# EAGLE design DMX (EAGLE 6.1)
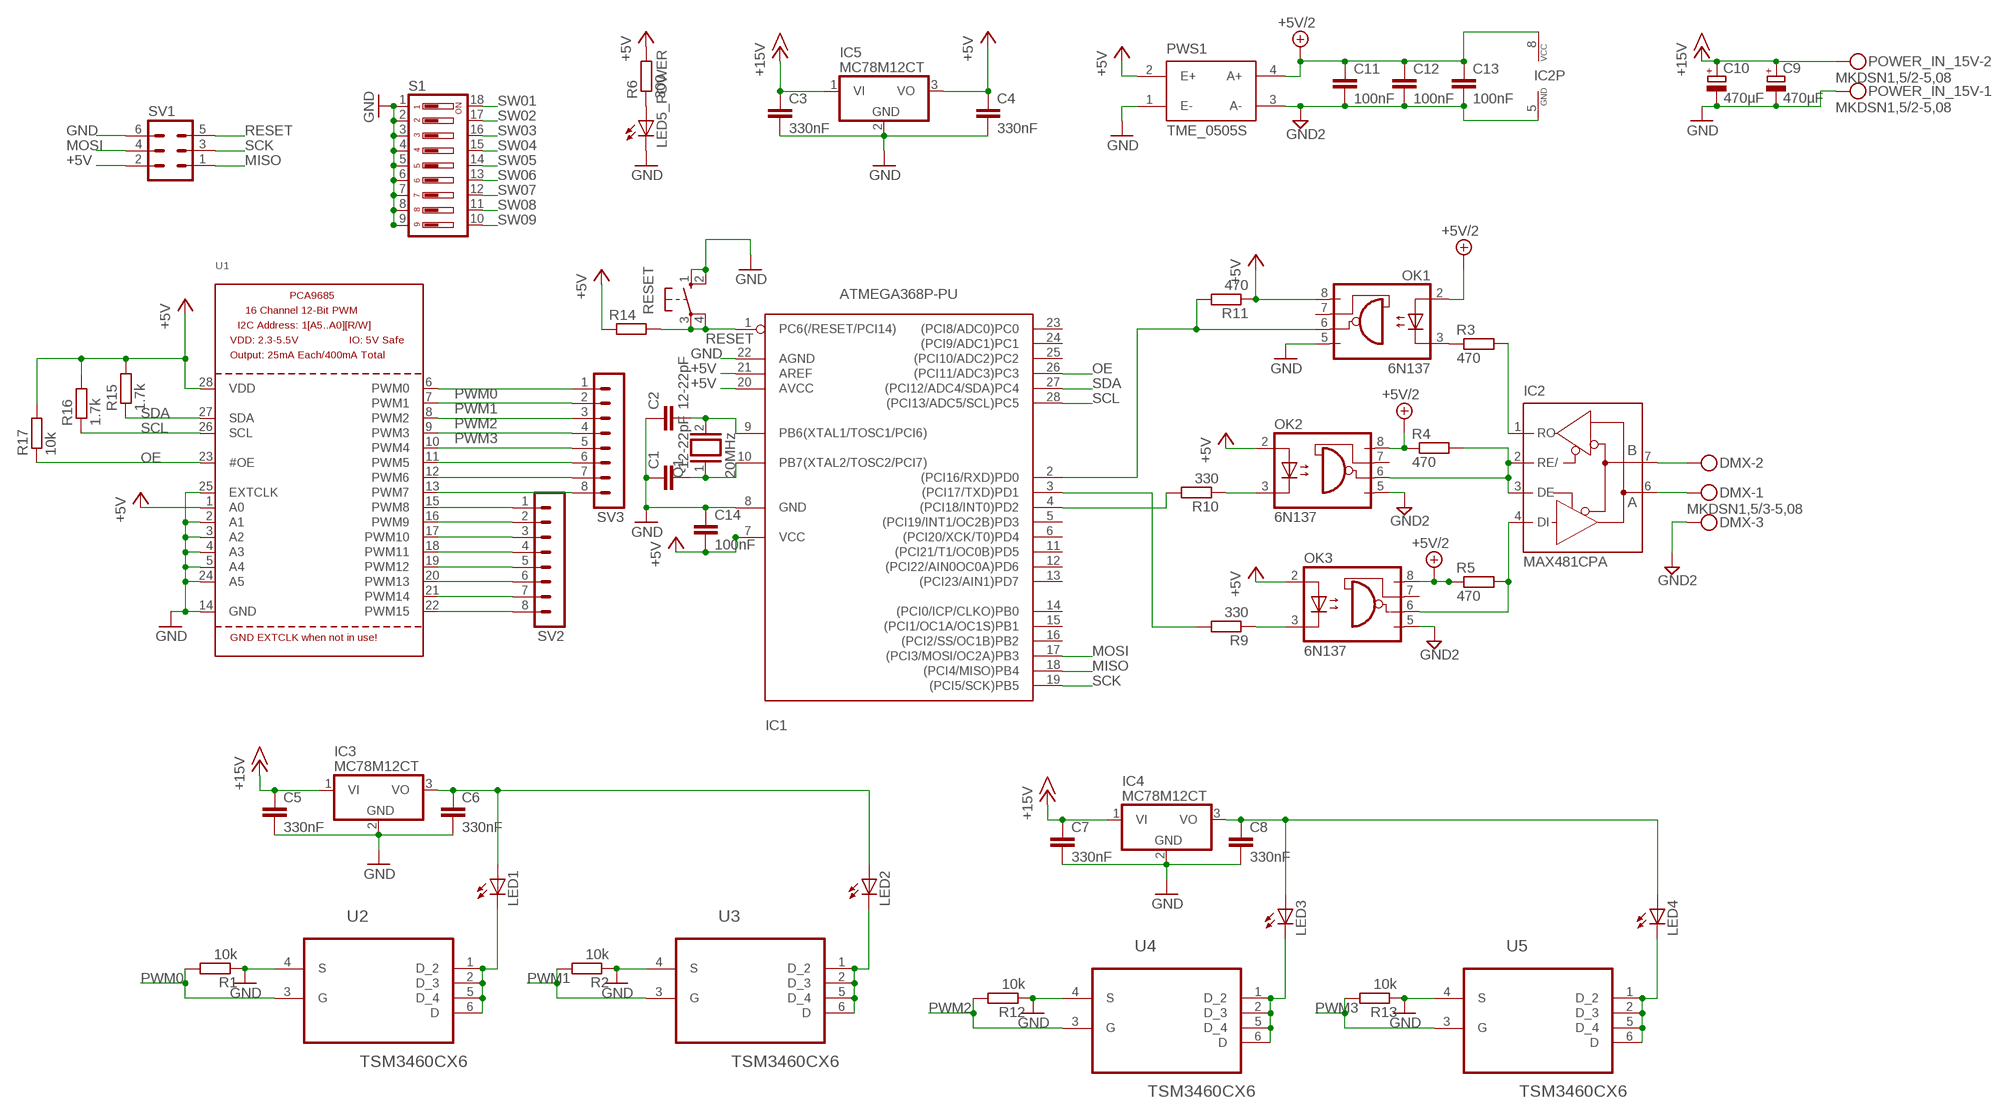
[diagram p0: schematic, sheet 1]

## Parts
C1  12-22pF  C-EU025-025X050  [C025-025X050]
C2  12-22pF  C-EU025-025X050  [C025-025X050]
C3  330nF  C-EU050-025X075  [C050-025X075]
C4  330nF  C-EU050-025X075  [C050-025X075]
C5  330nF  C-EU050-025X075  [C050-025X075]
C6  330nF  C-EU050-025X075  [C050-025X075]
C7  330nF  C-EU050-025X075  [C050-025X075]
C8  330nF  C-EU050-025X075  [C050-025X075]
C9  470µF  CPOL-EUE5-10.5  [E5-10,5]
C10  470µF  CPOL-EUE5-10.5  [E5-10,5]
C11  100nF  C-EU050-025X075  [C050-025X075]
C12  100nF  C-EU050-025X075  [C050-025X075]
C13  100nF  C-EU050-025X075  [C050-025X075]
C14  100nF  C-EU050-025X075  [C050-025X075]
DMX  MKDSN1,5/3-5,08  [MKDSN1,5/3-5,08]
IC1  ATMEGA368P-PU  ATMEGA168-20P  [DIL28-3]
IC2  MAX481CPA  [DIL08]
IC3  MC78M12CT  [TO220V]
IC4  MC78M12CT  [TO220V]
IC5  MC78M12CT  [TO220V]
LED1  LED5MM  [LED5MM]
LED2  LED5MM  [LED5MM]
LED3  LED5MM  [LED5MM]
LED4  LED5MM  [LED5MM]
LED5_POWER  LED5MM  [LED5MM]
OK1  6N137  [DIL08]
OK2  6N137  [DIL08]
OK3  6N137  [DIL08]
POWER_IN_15V  MKDSN1,5/2-5,08  [MKDSN1,5/2-5,08]
PWS1  TME_0505S  [TMEXXXXS]
Q1  20MHz  XTAL/S  [QS]
R1  10k  R-EU_0207/7  [0207/7]
R2  10k  R-EU_0207/7  [0207/7]
R3  470  R-EU_0207/7  [0207/7]
R4  470  R-EU_0207/7  [0207/7]
R5  470  R-EU_0207/7  [0207/7]
R6  300  R-EU_0204/7  [0204/7]
R9  330  R-EU_0207/7  [0207/7]
R10  330  R-EU_0207/7  [0207/7]
R11  470  R-EU_0207/7  [0207/7]
R12  10k  R-EU_0207/7  [0207/7]
R13  10k  R-EU_0207/7  [0207/7]
R14  R-EU_0204/7  [0204/7]
R15  1.7k  R-EU_0204/7  [0204/7]
R16  1.7k  R-EU_0204/7  [0204/7]
R17  10k  R-EU_0204/7  [0204/7]
RESET  10-XX  [B3F-10XX]
S1  DP09  [DP-09]
SV1  MA03-2  [MA03-2]
SV2  MA08-1  [MA08-1]
SV3  MA08-1  [MA08-1]
U1  PCA9685  [TSSOP28]
U2  TSM3460CX6  [SOT95P280X120-6N]
U3  TSM3460CX6  [SOT95P280X120-6N]
U4  TSM3460CX6  [SOT95P280X120-6N]
U5  TSM3460CX6  [SOT95P280X120-6N]

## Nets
+5V: C4.1 C14.2 IC1.7(VCC) IC1.20(AVCC) IC1.21(AREF) IC5.3(VO) OK1.8(VCC) OK2.2(A) OK3.2(A) PWS1.2(E+) R6.2 R11.1 R14.1 R15.2 R16.2 R17.2 SV1.2 U1.1(A0) U1.28(VDD)
+5V/2: C11.1 C12.1 C13.1 IC2.8(VCC) OK1.2(A) OK2.8(VCC) OK3.8(VCC) PWS1.4(A+) R4.1 R5.1
+15V: C3.1 C5.1 C7.1 C9.+ C10.+ IC3.1(VI) IC4.1(VI) IC5.1(VI) POWER_IN_15V.2
GND: C1.1 C2.1 C3.2 C4.2 C5.2 C6.2 C7.2 C8.2 C9.- C10.- C14.1 IC1.8(GND) IC1.22(AGND) IC3.2(GND) IC4.2(GND) IC5.2(GND) LED5_POWER.K(C) OK1.5(GND) POWER_IN_15V.1 PWS1.1(E-) R1.1 R2.1 R12.1 R13.1 RESET.1(S) RESET.2(S1) S1.1 S1.2 S1.3 S1.4 S1.5 S1.6 S1.7 S1.8 S1.9 SV1.6 U1.2(A1) U1.3(A2) U1.4(A3) U1.5(A4) U1.14(GND) U1.24(A5) U1.25(EXTCLK) U2.4(S) U3.4(S) U4.4(S) U5.4(S)
GND2: C11.2 C12.2 C13.2 DMX.3 IC2.5(GND) OK2.5(GND) OK3.5(GND) PWS1.3(A-)
MISO: IC1.18((PCI4/MISO)PB4) SV1.1
MOSI: IC1.17((PCI3/MOSI/OC2A)PB3) SV1.4
N$1: OK1.3(C) R3.1
N$2: IC2.1(RO) R3.2
N$3: IC2.2(RE/) IC2.3(DE) OK2.6(VO) R4.2
N$4: IC2.4(DI) OK3.6(VO) R5.2
N$5: OK3.3(C) R9.1
N$6: OK2.3(C) R10.1
N$7: IC1.2((PCI16/RXD)PD0) OK1.6(VO) R11.2
N$8: IC1.4((PCI18/INT0)PD2) R10.2
N$9: IC1.3((PCI17/TXD)PD1) R9.2
N$10: DMX.2 IC2.7(B)
N$11: DMX.1 IC2.6(A)
N$12: C6.1 IC3.3(VO) LED1.A LED2.A
N$13: LED3.K(C) U4.1(D_2) U4.2(D_3) U4.5(D_4) U4.6(D)
N$14: C8.1 IC4.3(VO) LED3.A LED4.A
N$15: LED1.K(C) U2.1(D_2) U2.2(D_3) U2.5(D_4) U2.6(D)
N$16: LED4.K(C) U5.1(D_2) U5.2(D_3) U5.5(D_4) U5.6(D)
N$17: LED2.K(C) U3.1(D_2) U3.2(D_3) U3.5(D_4) U3.6(D)
N$18: C1.2 IC1.10(PB7(XTAL2/TOSC2/PCI7)) Q1.1
N$19: C2.2 IC1.9(PB6(XTAL1/TOSC1/PCI6)) Q1.2
N$20: LED5_POWER.A R6.1
N$22: SV3.5 U1.10(PWM4)
N$23: SV3.6 U1.11(PWM5)
N$24: SV3.7 U1.12(PWM6)
N$25: SV3.8 U1.13(PWM7)
N$26: SV2.1 U1.15(PWM8)
N$27: SV2.2 U1.16(PWM9)
N$28: SV2.3 U1.17(PWM10)
N$29: SV2.4 U1.18(PWM11)
N$30: SV2.5 U1.19(PWM12)
N$31: SV2.6 U1.20(PWM13)
N$32: SV2.7 U1.21(PWM14)
N$33: SV2.8 U1.22(PWM15)
OE: IC1.26((PCI11/ADC3)PC3) R17.1 U1.23(#OE)
PWM0: R1.2 SV3.1 U1.6(PWM0) U2.3(G)
PWM1: R2.2 SV3.2 U1.7(PWM1) U3.3(G)
PWM2: R12.2 SV3.3 U1.8(PWM2) U4.3(G)
PWM3: R13.2 SV3.4 U1.9(PWM3) U5.3(G)
RESET: IC1.1(PC6(/RESET/PCI14)) R14.2 RESET.3(P) RESET.4(P1) SV1.5
SCK: IC1.19((PCI5/SCK)PB5) SV1.3
SCL: IC1.28((PCI13/ADC5/SCL)PC5) R16.1 U1.26(SCL)
SDA: IC1.27((PCI12/ADC4/SDA)PC4) R15.1 U1.27(SDA)
SW01: S1.18
SW02: S1.17
SW03: S1.16
SW04: S1.15
SW05: S1.14
SW06: S1.13
SW07: S1.12
SW08: S1.11
SW09: S1.10
Unconnected: IC1.5((PCI19/INT1/OC2B)PD3) IC1.6((PCI20/XCK/T0)PD4) IC1.11((PCI21/T1/OC0B)PD5) IC1.12((PCI22/AIN0OC0A)PD6) IC1.13((PCI23/AIN1)PD7) IC1.14((PCI0/ICP/CLKO)PB0) IC1.15((PCI1/OC1A/OC1S)PB1) IC1.16((PCI2/SS/OC1B)PB2) IC1.23((PCI8/ADC0)PC0) IC1.24((PCI9/ADC1)PC1) IC1.25((PCI10/ADC2)PC2) OK1.7(VE) OK2.7(VE) OK3.7(VE)

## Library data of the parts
C1-C8 C11-C14 = rcl:C-EU: CAPACITOR, European symbol
C9 C10 = rcl:CPOL-EU: POLARIZED CAPACITOR, European symbol
DMX = con-phoenix-508:MKDSN1,5/3-5,08: MKDSN 1,5/ 3-5,08 Printklemme Nennstrom: 13,5 A Nennspannung: 250 V Rastermaß: 5,08 mm Polzahl: 3 Anschlussart: Schraubanschluss Montage: Löten Anschlussrichtung Leiter/Platine: 0 ° Artikelnummer: 1729131 Source: http://eshop.phoenixcontact.com .. 1729131.pdf; MPN: SMKDSN1,5/3-5,08; OC_FARNELL: 1792904; OC_NEWARK: 70R0299
IC1 = adafruit:ATMEGA168*P: MICROCONTROLLER 16 kBytes FLASH 1 kBytes SRAM 512 Bytes EEPROM USART 8-channel 10 bit ADC
IC2 = maxim:MAX481CPA: RS485 TRANSEIVER; MPN: MAX485; OC_FARNELL: unknown; OC_NEWARK: 99K3445
IC3-IC5 = linear:MC78M: 500 mA Positive Voltage Regulators Source: Data sheet
LED1-LED4 LED5_POWER = led:LED: LED
OK1-OK3 = optocoupler:6N137: MOTOROLA OPTO COUPLER; MPN: 6N137; OC_FARNELL: 1328376; OC_NEWARK: 52M1895
POWER_IN_15V = con-phoenix-508:MKDSN1,5/2-5,08: MKDSN 1,5/ 2-5,08 Printklemme; MPN: MKDSN 1,5/2-5.08; OC_FARNELL: 1792903; OC_NEWARK: 30M2397
PWS1 = traco-electronic:TME_*S: DC/DC Konverter 1 Watt Source: http://www.tracopower.com/datasheet_g/tme-d.pdf; MPN: TME 0505S; OC_FARNELL: 1007538; OC_NEWARK: 51R5321
Q1 = special:XTAL/S: CRYSTAL
R1-R6 R9-R17 = rcl:R-EU_: RESISTOR, European symbol
RESET = switch-omron:10-XX: OMRON SWITCH; MPN: B3F-1000; OC_FARNELL: 176432; OC_NEWARK: 36M3542
S1 = switch-dil:DP09: DIL/CODE SWITCH; MPN: MCDP09; OC_FARNELL: 1522007; OC_NEWARK: 74M2979
SV1 = con-lstb:MA03-2: PIN HEADER; OC_FARNELL: unknown; OC_NEWARK: unknown
SV2 SV3 = con-lstb:MA08-1: PIN HEADER; OC_FARNELL: unknown; OC_NEWARK: unknown
U1 = adafruit:PCA9685: PCA9685 - 16 Channel 12-Bit I2C PWM Controller 5.0V tolerant 16 channel, 12-bit I2C PWM controller with 25mA per output (max. 400mA total) Digikey: 568-5931-1-ND
U2-U5 = farnell:TSM3460CX6: N-Channel MOSFET; MPN: TSM3460CX6; OC_FARNELL: 1864595; OC_NEWARK: 27T3007; PACKAGE: SOT-6; SUPPLIER: Taiwan Semiconductors

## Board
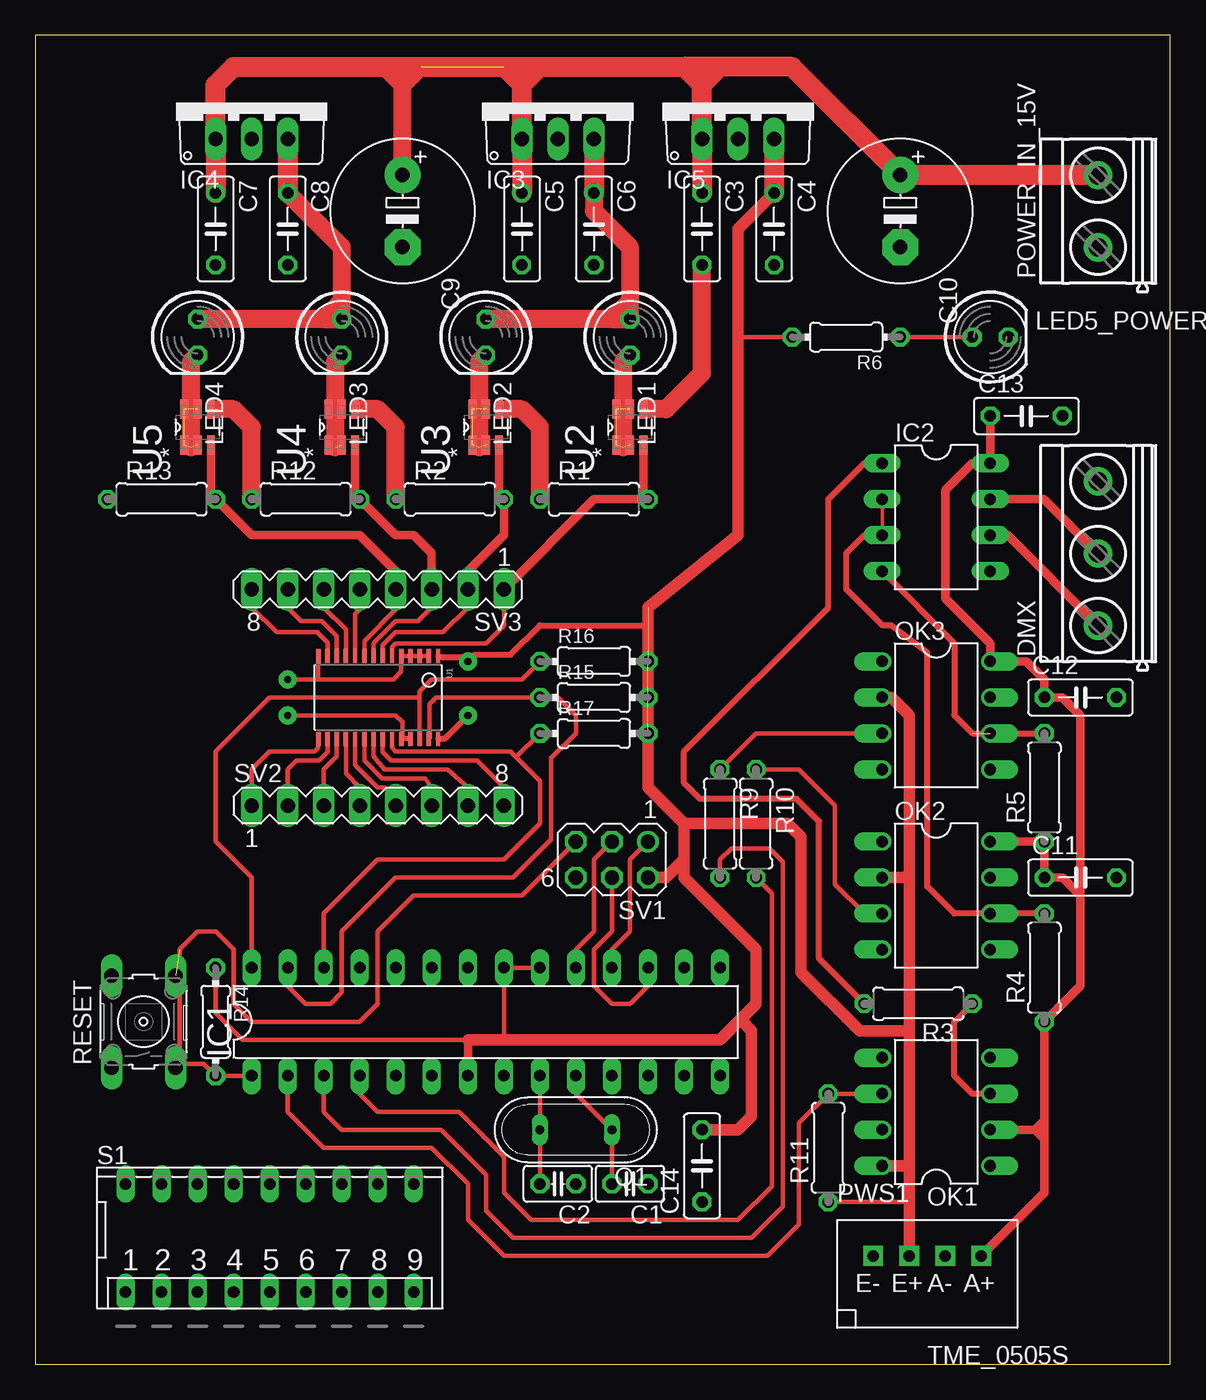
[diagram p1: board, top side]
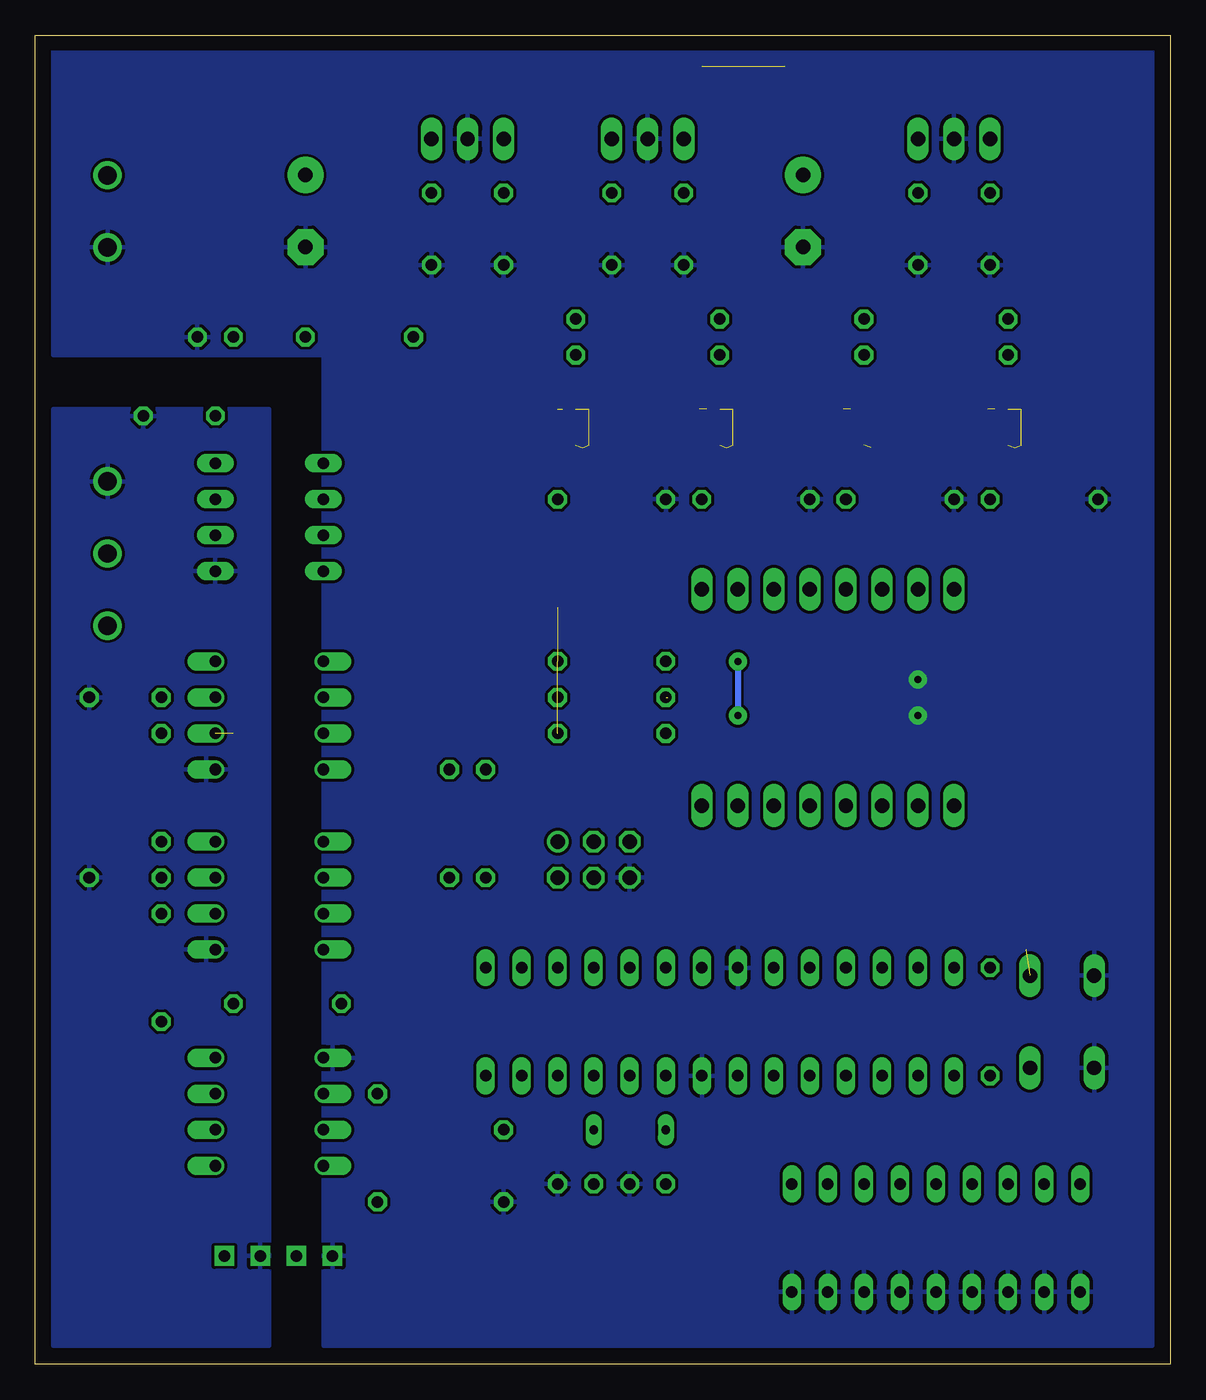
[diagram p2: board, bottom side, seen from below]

Size 79.99 x 93.65 mm. Coordinates in mm from the lower left corner, seen from the top.
Outline: 0,0 79.99,0 79.99,93.65 0,93.65 0,0
Copper layers (1*16): Top 0.035mm / dielectric 1.5mm / Bottom 0.035mm
Design rules: minimum track width 10mil, minimum drill 18mil, track to track 8mil, track to pad 8mil, pad to pad 8mil, via to via 8mil, smd to smd 8mil, copper to edge 40mil, drill to drill 8mil, minimum pad ring 10mil, minimum via ring 8mil, stop-mask expansion 4mil, vias tented up to drill 0mil, thermal gap 10mil

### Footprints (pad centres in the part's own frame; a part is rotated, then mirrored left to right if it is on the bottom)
C025-025X050 = drill 0.813 octagon: 1 -1.27,0; 2 1.27,0
C050-025X075 = drill 0.813 octagon: 1 -2.54,0; 2 2.54,0
E5-10,5 = drill 1.016 pad 2.54: + -2.54,0 | drill 1.016 pad 2.54 octagon: - 2.54,0
MKDSN1,5/3-5,08 = drill 1.3 pad 2: 1 -7.641,0.025; 2 -2.561,0.025; 3 2.519,0.025
DIL28-3 = drill 0.813 long: 1 -16.51,-3.81; 2 -13.97,-3.81; 3 -11.43,-3.81; 4 -8.89,-3.81; 5 -6.35,-3.81; 6 -3.81,-3.81; 7 -1.27,-3.81; 8 1.27,-3.81; 9 3.81,-3.81; 10 6.35,-3.81; 11 8.89,-3.81; 12 11.43,-3.81; 13 13.97,-3.81; 14 16.51,-3.81; 15 16.51,3.81; 16 13.97,3.81; 17 11.43,3.81; 18 8.89,3.81; 19 6.35,3.81; 20 3.81,3.81; 21 1.27,3.81; 22 -1.27,3.81; 23 -3.81,3.81; 24 -6.35,3.81; 25 -8.89,3.81; 26 -11.43,3.81; 27 -13.97,3.81; 28 -16.51,3.81
DIL08 = drill 0.813 long: 1 -3.81,-3.81; 2 -1.27,-3.81; 3 1.27,-3.81; 4 3.81,-3.81; 5 3.81,3.81; 6 1.27,3.81; 7 -1.27,3.81; 8 -3.81,3.81
TO220V = drill 1.016 long: 1 -2.54,-2.54; 2 0,-2.54; 3 2.54,-2.54
LED5MM = drill 0.813 octagon: A -1.27,0; K 1.27,0
DIL08' = drill 0.813 offset: 1 -3.81,-3.81; 2 -1.27,-3.81; 3 1.27,-3.81; 4 3.81,-3.81; 5 3.81,3.81; 6 1.27,3.81; 7 -1.27,3.81; 8 -3.81,3.81
MKDSN1,5/2-5,08 = drill 1.3 pad 2: 1 -2.561,0.025; 2 2.519,0.025
TMEXXXXS = drill 0.813 pad 1.397 square: 1 -3.81,1.27; 2 -1.27,1.27; 3 1.27,1.27; 4 3.81,1.27
QS = drill 0.61 long: 1 -2.54,0; 2 2.54,0
0207/7 = drill 0.813 octagon: 1 -3.81,0; 2 3.81,0
0204/7 = drill 0.813 octagon: 1 -3.81,0; 2 3.81,0
B3F-10XX = drill 1.016 long: 1 -3.251,2.261; 2 3.251,2.261; 3 -3.251,-2.261; 4 3.251,-2.261
DP-09 = drill 0.813 long: 1 -10.16,-3.81; 2 -7.62,-3.81; 3 -5.08,-3.81; 4 -2.54,-3.81; 5 0,-3.81; 6 2.54,-3.81; 7 5.08,-3.81; 8 7.62,-3.81; 9 10.16,-3.81; 10 10.16,3.81; 11 7.62,3.81; 12 5.08,3.81; 13 2.54,3.81; 14 0,3.81; 15 -2.54,3.81; 16 -5.08,3.81; 17 -7.62,3.81; 18 -10.16,3.81
MA03-2 = drill 1.016: 1 -2.54,-1.27 | drill 1.016 octagon: 2 -2.54,1.27; 3 0,-1.27; 4 0,1.27; 5 2.54,-1.27; 6 2.54,1.27
MA08-1 = drill 1.016 long: 1 -8.89,0; 2 -6.35,0; 3 -3.81,0; 4 -1.27,0; 5 1.27,0; 6 3.81,0; 7 6.35,0; 8 8.89,0
TSSOP28 = smd 0.305 x 0.991: 1 -4.225,-2.918; 2 -3.575,-2.918; 3 -2.925,-2.918; 4 -2.275,-2.918; 5 -1.625,-2.918; 6 -0.975,-2.918; 7 -0.325,-2.918; 8 0.325,-2.918; 9 0.975,-2.918; 10 1.625,-2.918; 11 2.275,-2.918; 12 2.925,-2.918; 13 3.575,-2.918; 14 4.225,-2.918; 15 4.225,2.918; 16 3.575,2.918; 17 2.925,2.918; 18 2.275,2.918; 19 1.625,2.918; 20 0.975,2.918; 21 0.325,2.918; 22 -0.325,2.918; 23 -0.975,2.918; 24 -1.625,2.918; 25 -2.275,2.918; 26 -2.925,2.918; 27 -3.575,2.918; 28 -4.225,2.918
SOT95P280X120-6N = smd 1.321 x 0.559: 1 -1.27,0.94; 2 -1.27,0; 3 -1.27,-0.94; 4 1.27,-0.94; 5 1.27,0; 6 1.27,0.94

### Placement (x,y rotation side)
C1  41.91,12.7 180 top
C2  36.83,12.7 180 top
C3  46.99,80.01 270 top
C4  52.07,80.01 270 top
C5  34.29,80.01 270 top
C6  39.37,80.01 270 top
C7  12.7,80.01 270 top
C8  17.78,80.01 270 top
C9  25.88,81.28 270 top
C10  60.96,81.28 270 top
C11  73.66,34.29 0 top
C12  73.66,46.99 0 top
C13  69.85,66.83 0 top
C14  46.99,13.97 90 top
DMX  74.93,59.69 90 top
IC1  31.75,24.13 0 top
IC2  63.5,59.69 270 top
IC3  36.83,88.9 0 top
IC4  15.24,88.9 0 top
IC5  49.53,88.9 0 top
LED1  41.91,72.39 270 top
LED2  31.75,72.39 270 top
LED3  21.59,72.39 270 top
LED4  11.43,72.39 270 top
LED5_POWER  67.31,72.39 0 top
OK1  6N137  [DIL08']  63.5,17.78 90 top
OK2  6N137  [DIL08']  63.5,33.02 270 top
OK3  6N137  [DIL08']  63.5,45.72 270 top
POWER_IN_15V  74.93,81.28 90 top
PWS1  62.87,6.35 0 top
Q1  38.1,16.51 180 top
R1  39.37,60.96 0 top
R2  29.21,60.96 0 top
R3  62.23,25.4 180 top
R4  71.12,27.94 90 top
R5  71.12,40.64 90 top
R6  57.15,72.39 180 top
R9  48.26,38.1 270 top
R10  50.8,38.1 270 top
R11  55.88,15.24 90 top
R12  19.05,60.96 0 top
R13  8.89,60.96 0 top
R14  12.7,24.13 270 top
R15  39.37,46.99 0 top
R16  39.37,49.53 0 top
R17  39.37,44.45 0 top
RESET  7.62,24.13 90 top
S1  16.51,8.89 0 top
SV1  40.64,35.56 180 top
SV2  24.13,39.37 0 top
SV3  24.13,54.61 180 top
U1  24.16,46.99 180 top
U2  41.91,66.04 90 top
U3  31.75,66.04 90 top
U4  21.59,66.04 90 top
U5  11.43,66.04 90 top

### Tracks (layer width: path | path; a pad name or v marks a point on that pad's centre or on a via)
+5V  (via drill 0.5 pad 1.27)  (4 unrouted)
  Top 0.305: R11.1 61.59,11.43 | R6.2 49.53,72.39 | IC1.20 IC1.21 33.02,22.86 30.48,22.86 14.61,22.86 12.7,24.77 R14.1
  Top 0.406: v30.48,45.72 28.83,44.07 U1.28 | U1.1 28.45,49.85 30.48,49.85 v30.48,49.53 30.96,50.01 33.5,50.01 35.56,52.07 43.18,52.07
  Top 0.61: IC1.7 30.48,22.86
  Top 0.813: C4.1 49.53,80.01 49.53,72.39 49.53,58.42 43.18,53.34 43.18,40.64 45.72,38.1 | PWS1.2 61.59,11.43 61.59,13.97 | 61.59,13.97 61.59,23.5 | 61.59,34.29 61.59,45.72 60.33,46.99 OK3.2 | OK1.8 61.59,13.97 | OK2.2 61.59,34.29 | 61.59,34.29 61.59,23.5 | 61.59,23.5 58.1,23.5 53.98,27.62 53.98,37.15 53.02,38.1 45.72,38.1 | 49.61,24.21 50.8,25.4 50.8,29.21 45.72,34.29 45.72,35.56 | 49.61,24.21 48.26,22.86 30.48,22.86 | 45.72,35.56 45.72,38.1 | SV1.2 44.45,34.29 45.72,35.56 | C14.2 49.53,16.51 50.48,17.46 50.48,23.5 49.77,24.21 49.61,24.21
  Top 1.422: IC5.3 C4.1
  Bottom 0.406: v30.48,49.53 v30.48,45.72
+5V/2
  Top 0.61: PWS1.4 71.12,12.06 71.12,15.88 | 71.12,15.88 70.48,16.51 | OK1.2 70.48,16.51 | 70.48,16.51 71.12,17.14 | 71.12,17.14 71.12,15.88 | 71.12,17.14 R4.1 73.66,26.67 73.66,33.02 | OK2.8 R5.1 C11.1 72.39,34.29 73.66,33.02 | C13.1 IC2.8 66.04,63.5 64.14,61.59 64.14,53.98 67.31,50.8 OK3.8 69.85,49.53 71.12,48.26 C12.1 72.39,46.99 73.66,45.72 73.66,33.02
+15V  (1 unrouted)
  Top 1.27: 60.98,83.8 C10.+ | C9.+ 25.88,90.17 | 25.88,90.17 24.61,91.44 | 27.15,91.44 25.88,90.17
  Top 1.422: 48.26,91.44 45.72,91.44 | 45.72,91.44 46.99,90.17 | 46.99,90.17 IC5.1 C3.1 | 46.99,90.17 48.26,91.44 | 34.29,90.17 IC3.1 C5.1 | 34.29,90.17 33.02,91.44 35.56,91.44 34.29,90.17 | 45.72,91.44 27.15,91.44 24.61,91.44 13.97,91.44 12.7,90.17 IC4.1 C7.1 | POWER_IN_15V.2 60.98,83.8 | C10.+ 53.34,91.44 48.26,91.44
GND  (via drill 0.5 pad 1.27)  (4 unrouted)
  Top 0.305: U1.2 U1.3 U1.4 U1.5 25.79,48.8 25.24,48.26 19.84,48.26 | U1.24 U1.25 26.38,44.13 25.88,44.13 25.88,45.24 25.4,45.72 v17.78,45.72 | 19.84,48.26 v17.78,48.26 | U1.14 19.93,48.35 19.84,48.26
  Top 1.27: R12.1 15.24,66.04 13.97,67.31 12.86,67.31 | R2.1 25.4,66.04 24.13,67.31 23.02,67.31 | R1.1 35.56,66.04 34.29,67.31 33.18,67.31 | C3.2 46.99,69.85 44.45,67.31 43.18,67.31
  pour Bottom: 1.27,1.27 1.27,92.71 78.74,92.71 78.74,71.12 59.69,71.12 59.69,1.27
GND2
  pour Bottom: 63.5,1.27 63.5,67.31 78.74,67.31 78.74,1.27
MISO
  Top 0.305: SV1.1 41.91,35.56 41.91,30.48 40.64,29.21 IC1.18
MOSI
  Top 0.305: SV1.4 40.64,30.48 39.37,29.21 39.37,26.67 40.64,25.4 41.91,25.4 43.18,26.67 IC1.17
N$1
  Top 0.406: OK1.3 66.04,19.05 64.77,20.32 64.77,24.13 R3.1
N$2
  Top 0.406: R3.2 55.24,28.57 55.24,38.26 53.66,39.85 46.83,39.85 45.72,40.96 45.72,43.18 55.88,53.34 55.88,60.96 58.42,63.5 IC2.1
N$3
  Top 0.254: IC2.3 IC2.2
  Top 0.406: R4.2 OK2.6 64.77,31.75 62.87,33.66 62.87,50.16 60.33,52.07 59.69,52.07 57.15,54.61 57.15,57.15 58.42,58.42 IC2.3
N$4  (1 unrouted)
  Top 0.406: IC2.4 64.77,50.8 64.77,45.72 66.04,44.45 R5.2
N$5
  Top 0.305: R9.1 50.8,44.45 OK3.3
N$6
  Top 0.305: OK2.3 58.42,31.75 56.36,33.81 56.36,39.37 53.82,41.91 R10.1
N$7
  Top 0.305: IC1.2 17.78,17.78 20.32,15.24 27.94,15.24 30.48,12.7 30.48,10.16 33.02,7.62 51.59,7.62 53.82,9.84 53.82,16.99 R11.2 OK1.6
N$8
  Top 0.305: IC1.4 22.86,19.05 24.13,17.78 29.84,17.78 33.02,14.61 33.02,12.06 34.92,10.16 49.53,10.16 51.91,12.54 51.91,33.18 R10.2
N$9
  Top 0.305: IC1.3 20.32,17.78 21.59,16.51 28.57,16.51 31.75,13.34 31.75,10.79 33.66,8.89 50.48,8.89 52.7,11.11 52.7,35.4 51.75,36.35 49.05,36.35 48.26,35.56 R9.2
N$10
  Top 0.61: IC2.7 71.07,60.96 DMX.2
N$11
  Top 0.61: IC2.6 68.53,58.42 DMX.1
N$12
  Top 1.27: C6.1 39.37,81.28 41.91,78.74 41.91,74.93 | 41.91,74.93 40.64,73.66 | 40.64,73.66 LED1.A 41.91,74.93 | 40.64,73.66 LED2.A
  Top 1.422: IC3.3 C6.1
N$13  (1 unrouted)
  Top 0.305: U4.2 U4.1 U4.6 U4.5
  Top 1.27: LED3.K 21.11,70.64 21.11,64.61
N$14
  Top 1.27: C8.1 21.59,78.74 21.59,74.93 | LED3.A 21.59,74.93 | 21.59,74.93 20.32,73.66 LED3.A | LED3.A LED4.A
  Top 1.422: IC4.3 C8.1
N$15  (4 unrouted)
  Top 1.27: LED1.K 41.43,70.64 41.43,64.61
N$16  (4 unrouted)
  Top 1.27: LED4.K 10.95,70.64 10.95,64.61
N$17  (4 unrouted)
  Top 1.27: LED2.K 31.27,70.64 31.27,64.61
N$18
  Top 0.305: IC1.10 38.1,19.05 Q1.1 C1.2
N$19
  Top 0.305: IC1.9 Q1.2 C2.2
N$20
  Top 0.305: R6.1 LED5_POWER.A
N$22
  Top 0.305: U1.10 22.54,52.86 22.86,53.18 SV3.5
N$23
  Top 0.305: U1.11 21.89,51.77 20.32,53.34 SV3.6
N$24
  Top 0.305: U1.12 21.23,51.31 20.16,52.39 18.73,52.39 17.78,53.34 SV3.7
N$25
  Top 0.305: U1.13 20.59,50.85 19.84,51.59 16.99,51.59 15.24,53.34 SV3.8
N$26
  Top 0.305: U1.15 19.93,43.43 19.68,43.18 16.51,43.18 15.24,41.91 SV2.1
N$27
  Top 0.305: U1.16 20.59,43.13 20,42.55 18.41,42.55 17.78,41.91 SV2.2
N$28
  Top 0.305: U1.17 21.23,42.83 20.32,41.91 SV2.3
N$29
  Top 0.305: U1.18 21.89,41.62 22.86,40.64 SV2.4
N$30
  Top 0.305: U1.19 22.54,42.23 24.13,40.64 24.61,40.64 25.4,39.85 SV2.5
N$31
  Top 0.305: U1.20 23.18,42.54 24.45,41.27 27.46,41.27 27.94,40.64 SV2.6
N$32
  Top 0.305: U1.21 23.84,42.84 24.61,41.91 29.05,41.91 30.48,40.64 SV2.7
N$33
  Top 0.305: U1.22 24.48,43.14 25.08,42.55 31.11,42.55 33.02,40.64 SV2.8
OE
  Top 0.305: U1.23 25.14,43.45 25.4,43.18 33.5,43.18 33.89,42.78 | 33.89,42.78 35.56,41.12 35.56,38.1 33.02,35.56 24.13,35.56 20.32,31.75 IC1.26 | R17.1 33.89,42.78
PWM0
  Top 0.305: U1.6 25.14,50.53 25.4,50.8 31.75,50.8 33.02,52.07 SV3.1
  Top 0.61: U2.3 42.85,61.29 R1.2 39.37,60.96 SV3.1
PWM1
  Top 0.305: U1.7 24.48,50.68 25.4,51.59 28.73,51.59 30.48,53.34 SV3.2
  Top 0.61: U3.3 32.69,61.29 R2.2 33.02,58.42 30.48,55.88 SV3.2
PWM2
  Top 0.305: U1.8 23.84,50.82 25.4,52.39 26.99,52.39 27.94,53.34 SV3.3
  Top 0.61: U4.3 22.53,61.29 R12.2 25.4,58.42 26.67,58.42 27.94,57.15 SV3.3
PWM3
  Top 0.305: U1.9 23.18,50.97 25.4,53.18 SV3.4
  Top 0.61: U5.3 12.37,61.29 R13.2 15.24,58.42 22.86,58.42 25.4,55.88 SV3.4
RESET  (1 unrouted)
  Top 0.305: SV1.5 34.29,33.02 26.67,33.02 24.13,30.48 24.13,25.4 22.86,24.13 15.24,24.13 13.97,25.4 13.97,29.21 12.7,30.48 11.43,30.48 10.16,29.21 10.16,21.16 | 10.16,21.16 RESET.3 | 10.16,21.16 11.86,21.16 R14.2 IC1.1
SCK
  Top 0.305: SV1.3 39.37,35.56 39.37,30.48 38.1,29.21 IC1.19
SCL
  Top 0.305: IC1.28 15.24,34.29 12.7,36.83 12.7,43.18 16.51,46.99 27.09,46.99 | R16.1 34.29,48.26 27.94,48.26 27.09,47.41 27.09,46.99 | U1.26 27.09,46.99
SDA  (1 unrouted)
  Top 0.305: R15.1 36.83,46.99 38.1,45.72 38.1,44.45 36.35,42.7 36.35,36.99 33.66,34.29 25.4,34.29 21.59,30.48 21.59,26.19 20.8,25.4 19.05,25.4 17.78,26.67 IC1.27 | U1.27 27.78,44.12 27.78,46.51 28.26,46.99 35.4,46.99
